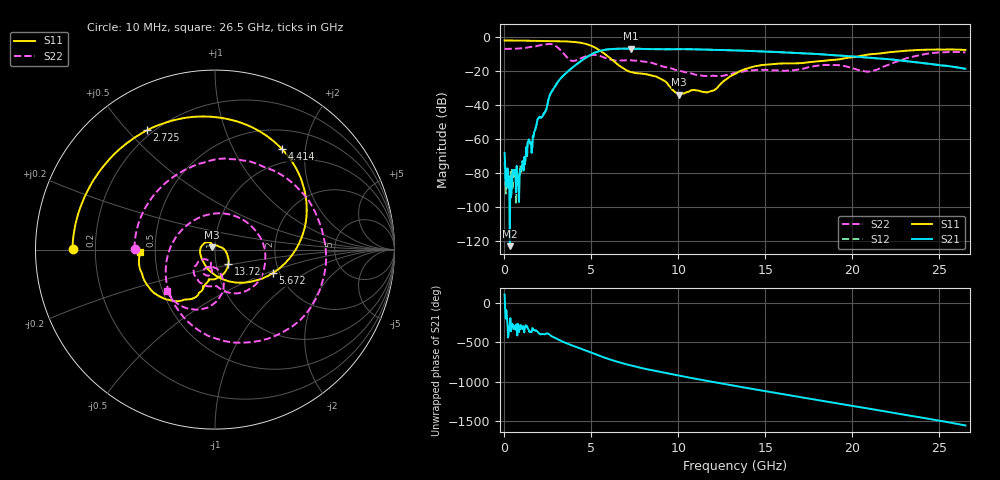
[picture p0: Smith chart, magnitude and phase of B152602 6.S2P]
!  2-Port S-parameters saved by WinCal
! VAR MeasName=S-Parameters (CALIBRATED_DATA) read from VNA (N5242A)
! VAR MeasDate=2016-1-5 16:26:26
! VAR NAME=B152602 6
! VAR FILENAME=B152602 6.S2P
! VAR DATE=2016-1-5 16:26:26
! VAR PHYS_PORTS=1,2
# Hz S DB R 50
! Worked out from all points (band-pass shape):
!   801 points, 10 MHz to 26.5 GHz, reference 50 ohm
!   highest |S21| = -6.78 dB at 7.262 GHz (marker M1); lowest = -122.8 dB at 308 MHz (marker M2)
!   |S21| within 3 dB of the highest: 5.07 GHz to 17.65 GHz (12.58 GHz wide, 111 % of centre)
!   lowest |S11| = -33.7 dB at 10.04 GHz (marker M3), VSWR 1.04, Z = 48.4 + j1.26 ohm
!   |S11| at or under -10 dB: 5.78 GHz to 21.17 GHz (15.39 GHz wide, 114 % of centre)
!   |S22| runs from -23.1 to -4.1 dB; largest |S21 - S12| = 0.0029
!   S11 on the Smith chart (normalised r, x): 10 MHz: 0.11, +0.00; 2.725 GHz: 0.18, +0.57; 4.414 GHz: 0.77, +1.58; 5.672 GHz: 1.84, -0.55; 13.72 GHz: 1.15, -0.18; 26.5 GHz: 0.41, -0.02
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1e7  -2.01 179.8  -68.13 103.5  -73.27 4.7  -6.97 179.4
3.080125e8  -2.03 173.6  -122.78 49.1  -85.37 137.9  -6.93 161.1
8.378125e8  -2.09 162.8  -96.87 -12.8  -82.51 46.4  -6.71 128.1
1.73185e9  -2.20 143.9  -55.37 15.2  -55.62 13.4  -5.50 65.0
2.360988e9  -2.28 129.3  -43.56 -38.7  -43.52 -38.6  -4.31 6.8
2.725225e9  -2.32 119.7  -31.95 -66.9  -31.99 -67.0  -4.21 -39.9
3.023238e9  -2.39 111.2  -27.02 -98.9  -27.03 -98.9  -5.81 -84.1
3.420588e9  -2.52 98.6  -22.35 -140.5  -22.37 -140.5  -9.88 -148.1
4.413962e9  -3.43 56.6  -13.98 135.3  -13.99 135.4  -12.38 33.6
4.447075e9  -3.49 54.9  -13.74 132.6  -13.75 132.7  -12.24 29.6
5.672238e9  -9.19 -22.2  -7.69 29.9  -7.69 30.1  -11.81 -70.1
7.261638e9  -20.53 -134.4  -6.78 -75.3  -6.78 -75.3  -13.65 -105.0
8.851038e9  -23.83 141.5  -7.11 -153.2  -7.11 -153.2  -16.44 -139.8
1.004309e10  -33.74 140.7  -7.11 155.4  -7.10 155.4  -19.67 -144.1
1.19305e10  -31.60 50.2  -7.51 77.0  -7.51 76.9  -22.75 -122.0
1.3255e10  -21.65 -29.9  -7.84 25.2  -7.84 25.2  -21.04 -104.9
1.371858e10  -19.27 -46.4  -8.01 7.2  -7.99 7.2  -20.20 -104.4
1.577155e10  -15.56 -93.2  -8.84 -70.7  -8.84 -70.7  -19.59 -109.3
1.769208e10  -14.58 -103.1  -9.81 -142.7  -9.78 -142.6  -17.30 -98.8
2.01424e10  -11.72 -110.2  -11.48 126.4  -11.45 126.4  -18.74 -117.3
2.209604e10  -8.95 -126.2  -13.04 53.7  -12.96 53.4  -16.24 -75.3
2.65e10  -7.57 -177.8  -18.64 -116.5  -18.67 -116.7  -9.04 -138.8
